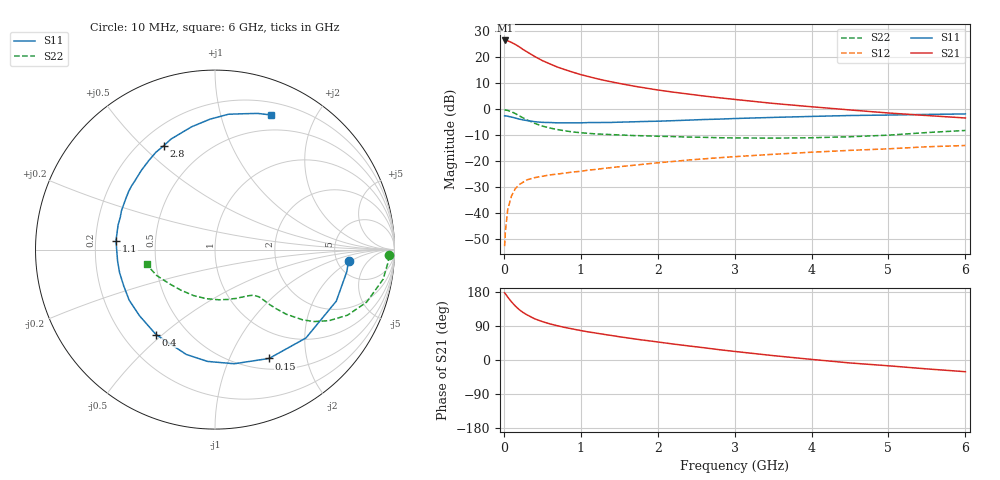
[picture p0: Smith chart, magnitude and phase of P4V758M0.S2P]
! SIEMENS Small Signal Semiconductors
! BFP182
! Si NPN RF Bipolar Junction Transistor in SOT143
! VCE = 0.75 V  IC = 8 mA
! Common Emitter S-Parameters:  March  1996
# GHz  S  MA  R  50
!  f  S11  S21  S12  S22
! GHz  MAG  ANG  MAG  ANG  MAG  ANG  MAG  ANG
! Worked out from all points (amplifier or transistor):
!   36 points, 10 MHz to 6 GHz, reference 50 ohm
!   highest |S21| = 26.5 dB at 20 MHz (marker M1)
!   |S21| within 3 dB of that: start of sweep to 226.9 MHz
!   unconditionally stable (mu >= 1): 1.007 GHz to end of sweep
!   at 250 MHz: K = 0.33, MSG = 25.6 dB, |S12| = -28.1 dB
!   at 1.4 GHz: K = 1.16, MAG = 14.1 dB, |S12| = -22.5 dB
!   at 6 GHz: K = 1.06, MAG = 3.8 dB, |S12| = -14.0 dB
!   S11 on the Smith chart (normalised r, x): 10 MHz: 6.40, -1.77; 150 MHz: 0.63, -1.42; 400 MHz: 0.34, -0.48; 1.1 GHz: 0.29, +0.04; 2.8 GHz: 0.29, +0.58; 6 GHz: 0.33, +1.45
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0.01  0.7468 -4.7  21.07 177.4  0.0023 83.6  0.9702 -1.9
0.02  0.7445 -9.5  21.17 174.9  0.0044 81.9  0.9676 -4.0
0.05  0.7343 -23.0  20.89 166.1  0.0116 80.6  0.9512 -10.0
0.1  0.7065 -44.2  19.36 153.4  0.0215 67.9  0.8942 -19.1
0.15  0.6771 -63.6  17.71 142.2  0.0296 60.0  0.8242 -26.3
0.2  0.645 -80.4  15.96 132.9  0.0353 54.2  0.7491 -31.9
0.25  0.6244 -93.8  14.2 125.4  0.0393 49.4  0.6819 -36.0
0.3  0.6057 -105.3  12.79 119.3  0.0436 45.5  0.6256 -38.7
0.4  0.5761 -124.8  10.43 108.8  0.0481 41.3  0.5358 -42.2
0.5  0.5593 -138.8  8.675 101.3  0.0511 38.5  0.4747 -44.0
0.6  0.555 -149.5  7.474 95.3  0.0544 37.7  0.4347 -45.1
0.7  0.5472 -158.4  6.469 90.2  0.0565 37.1  0.4051 -45.7
0.9  0.5465 -173.1  5.161 81.7  0.0619 37.2  0.3653 -46.8
1.1  0.5538 174.8  4.266 74.1  0.0673 37.3  0.3434 -48.6
1.5  0.5641 157.6  3.149 61.4  0.078 37.6  0.3203 -53.2
1.8  0.58 146.0  2.627 52.8  0.0867 38.0  0.3088 -57.9
2.2  0.6022 133.1  2.139 42.2  0.0986 36.5  0.2979 -65.7
2.8  0.6454 116.3  1.666 27.2  0.1165 33.2  0.2828 -79.9
3.5  0.6965 100.8  1.297 11.6  0.1355 28.5  0.2778 -99.9
4.5  0.7579 84.3  0.97 -7.8  0.1614 21.0  0.2954 -130.1
5.5  0.7952 72.6  0.757 -23.5  0.1892 13.8  0.3558 -156.1
6  0.8129 67.3  0.679 -30.9  0.2003 9.0  0.3902 -167.8
